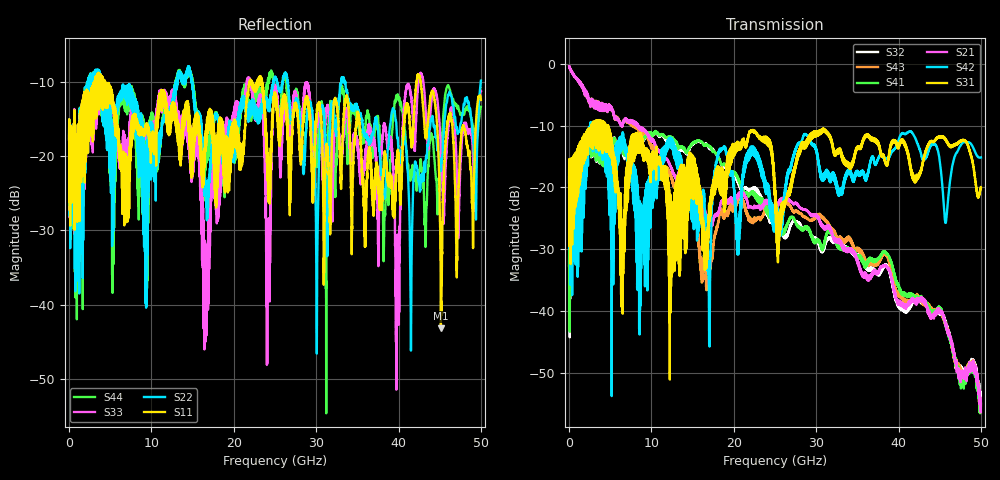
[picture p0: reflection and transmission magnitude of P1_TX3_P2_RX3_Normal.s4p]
!Keysight Technologies,N5225A,MY51441389,A.10.49.11
!Date: Monday, July 08, 2019 11:16:27
!Correction: S11(Full 4 Port(1,2,3,4))
!S12(Full 4 Port(1,2,3,4))
!S13(Full 4 Port(1,2,3,4))
!S14(Full 4 Port(1,2,3,4))
!S21(Full 4 Port(1,2,3,4))
!S22(Full 4 Port(1,2,3,4))
!S23(Full 4 Port(1,2,3,4))
!S24(Full 4 Port(1,2,3,4))
!S31(Full 4 Port(1,2,3,4))
!S32(Full 4 Port(1,2,3,4))
!S33(Full 4 Port(1,2,3,4))
!S34(Full 4 Port(1,2,3,4))
!S41(Full 4 Port(1,2,3,4))
!S42(Full 4 Port(1,2,3,4))
!S43(Full 4 Port(1,2,3,4))
!S44(Full 4 Port(1,2,3,4))
!S4P File: Measurements: <S11,S12,S13,S14>,
!<S21,S22,S23,S24>,
!<S31,S32,S33,S34>,
!<S41,S42,S43,S44>:
# Hz S  dB  R 50
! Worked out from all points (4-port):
!   5000 points, 10 MHz to 50 GHz, reference 50 ohm
!   strongest paths, dB at 10 MHz, 12.51 GHz, 25.01 GHz, 37.51 GHz, 50 GHz:
!     S31: -19.1, -23.2, -20.8, -12.6, -20.0
!     S42: -19.3, -12.2, -26.7, -15.4, -15.2
!     S21: -0.4, -17.0, -24.5, -33.8, -56.4
!     S41: -32.7, -12.0, -23.0, -31.7, -55.6
!     S43: -0.4, -18.6, -24.6, -32.3, -55.2
!     S32: -32.7, -12.4, -24.3, -34.2, -55.0
!   lowest |S11| = -43.2 dB at 45.14 GHz (marker M1), VSWR 1.01, Z = 49.4 - j0.402 ohm
!   |S11| at or under -10 dB: 4.381 GHz to 21.92 GHz (17.54 GHz wide, 133 % of centre); 23.42 GHz to 42.16 GHz (18.74 GHz wide, 57.2 % of centre); 42.67 GHz to end of sweep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
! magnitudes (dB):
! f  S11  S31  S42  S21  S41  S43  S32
! 10 MHz  -17.6  -19.1  -19.3  -0.4  -32.7  -0.4  -32.7
! 10.54 GHz  -15.9  -15.3  -16.7  -13.8  -10.9  -15.1  -11.0
! 16.62 GHz  -17.5  -28.8  -29.1  -24.3  -13.1  -34.4  -12.9
! 21.78 GHz  -11.2  -11.7  -14.4  -23.2  -21.5  -24.8  -20.6
! 24.17 GHz  -25.2  -13.1  -21.1  -22.2  -23.8  -23.1  -24.3
! 45.14 GHz  -43.2  -11.7  -17.2  -40.4  -40.2  -40.2  -40.5
! 50 GHz  -12.4  -20.0  -15.2  -56.4  -55.6  -55.2  -55.0
